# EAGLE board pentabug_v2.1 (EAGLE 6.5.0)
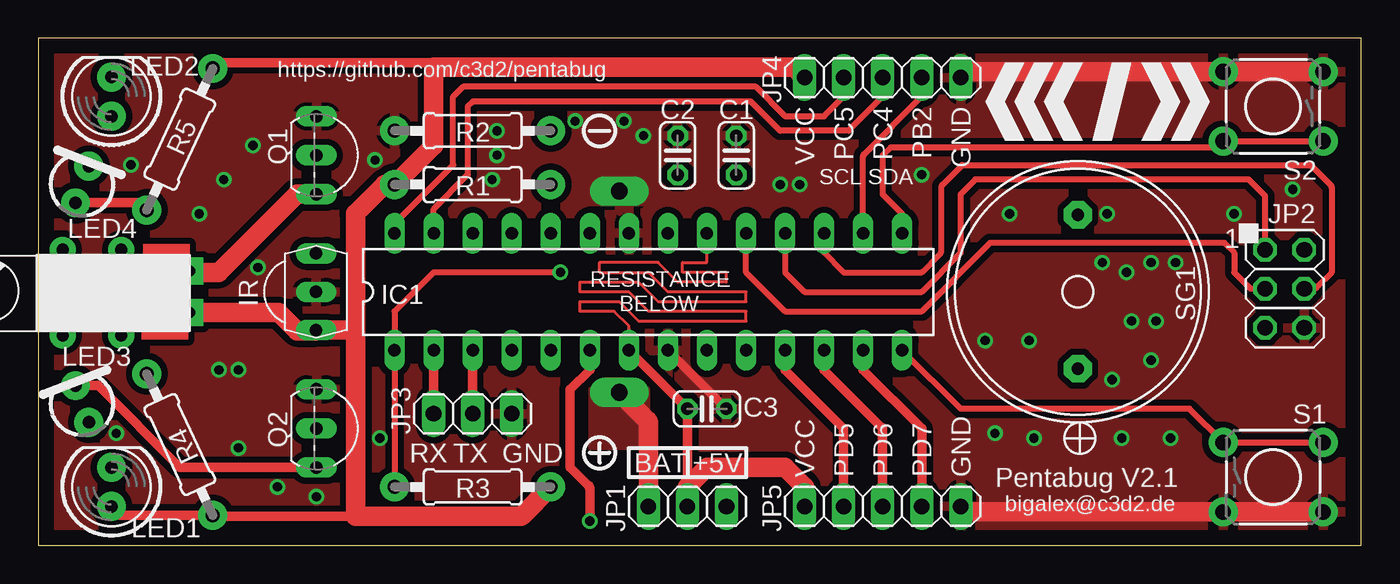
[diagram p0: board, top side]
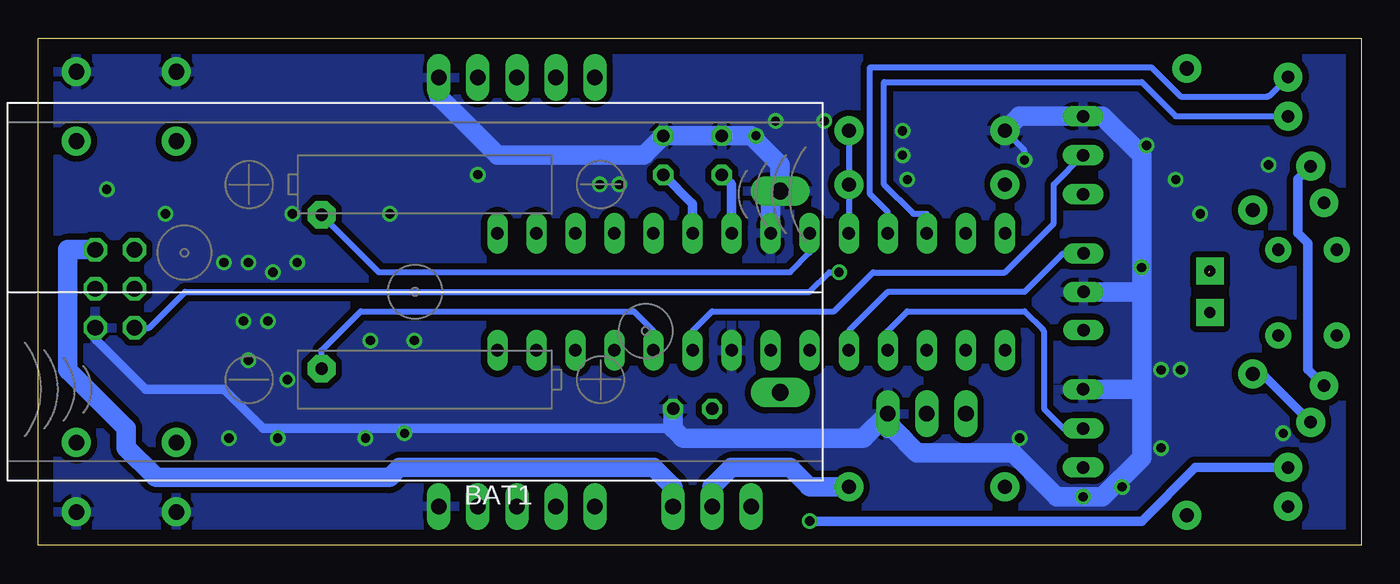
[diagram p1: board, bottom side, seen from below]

Size 86.03 x 33 mm. Coordinates in mm from the lower left corner, seen from the top.
Outline: 86.03,0 86.03,33 0,33 0,0 86.03,0
Copper layers (1*16): Top 0.035mm / dielectric 1.5mm / Bottom 0.035mm
Design rules "default *": minimum track width 8mil, minimum drill 0.6mm, track to track 8mil, track to pad 8mil, pad to pad 8mil, via to via 8mil, smd to smd 8mil, copper to edge 40mil, drill to drill 8mil, minimum pad ring 10mil, minimum via ring 8mil, stop-mask expansion 4mil, vias tented up to drill 0.8mm, thermal gap 10mil

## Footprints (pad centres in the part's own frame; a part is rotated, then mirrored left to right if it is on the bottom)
BATTERY_2XAAA_SMALLPINS = drill 1.1 pad 1.905 long: + -23.75,6.55; - -23.75,-6.55
C025-024X044 = drill 0.813 octagon: 1 -1.27,0; 2 1.27,0
DIL28-3 = drill 0.813 long: 1 -16.51,-3.81; 2 -13.97,-3.81; 3 -11.43,-3.81; 4 -8.89,-3.81; 5 -6.35,-3.81; 6 -3.81,-3.81; 7 -1.27,-3.81; 8 1.27,-3.81; 9 3.81,-3.81; 10 6.35,-3.81; 11 8.89,-3.81; 12 11.43,-3.81; 13 13.97,-3.81; 14 16.51,-3.81; 15 16.51,3.81; 16 13.97,3.81; 17 11.43,3.81; 18 8.89,3.81; 19 6.35,3.81; 20 3.81,3.81; 21 1.27,3.81; 22 -1.27,3.81; 23 -3.81,3.81; 24 -6.35,3.81; 25 -8.89,3.81; 26 -11.43,3.81; 27 -13.97,3.81; 28 -16.51,3.81
TSOP382 = drill 0.813 long: GND -0.001,-0.027; OUT -2.501,-0.027; VCC 2.499,-0.027
1X03 = drill 1.016 long: 1 -2.54,0; 2 0,0; 3 2.54,0
2X03 = drill 1.016 octagon: 1 -2.54,-1.27; 2 -2.54,1.27; 3 0,-1.27; 4 0,1.27; 5 2.54,-1.27; 6 2.54,1.27
1X05 = drill 1.016 long: 1 -5.08,0; 2 -2.54,0; 3 0,0; 4 2.54,0; 5 5.08,0
LED5MM = drill 0.813 pad 1.88: A -1.27,0; K 1.27,0
LED3MM = drill 0.813 pad 1.88: A -1.27,0; K 1.27,0
TO92- = drill 0.813 long: 1 -2.54,0; 2 0,0; 3 2.54,0
0207/10 = drill 0.914 pad 1.88: 1 -5.08,0; 2 5.08,0
TACTILE-PTH = drill 1.016 pad 1.88: 1 -3.251,2.261; 2 3.251,2.261; 3 -3.251,-2.261; 4 3.251,-2.261
BUZZRTDK = drill 0.8 pad 1.8 octagon: + 5,0; - -5,0
LA4-432 = drill 0.7 pad 1.778 square: P$1 -6.985,1.35; P$2 -6.985,-1.35

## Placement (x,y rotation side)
BAT1  BATTERY_2XAAA  [BATTERY_2XAAA_SMALLPINS]  61.53,16.51 180 bottom
C1  100nF  [C025-024X044]  45.39,25.4 270 top
C2  100nF  [C025-024X044]  41.58,25.4 270 top
C3  100nF  [C025-024X044]  43.48,8.89 180 top
IC1  ATMEGA328P-PU  [DIL28-3]  39.67,16.51 0 top
IR  TSOP382  [TSOP382]  18.09,16.51 270 top
JP1  [1X03]  42.21,2.54 180 top
JP2  [2X03]  81.07,16.71 270 top
JP3  [1X03]  28.25,8.57 0 top
JP4  [1X05]  54.91,30.45 0 top
JP5  [1X05]  54.91,2.54 0 top
LED1  [LED5MM]  4.75,3.81 90 top
LED2  [LED5MM]  4.75,29.21 90 top
LED3  [LED3MM]  2.85,9.21 110 top
LED4  [LED3MM]  2.85,23.5 70 top
Q1  [TO92-]  18.09,25.4 270 top
Q2  [TO92-]  18.09,7.62 270 top
R1  100K  [0207/10]  28.25,23.5 0 top
R2  22K  [0207/10]  28.25,26.99 180 top
R3  10k  [0207/10]  28.25,3.81 0 top
R4  33R  [0207/10]  9.2,6.57 295 top
R5  33R  [0207/10]  9.2,26.44 65 top
S1  [TACTILE-PTH]  80.31,4.45 0 top
S2  [TACTILE-PTH]  80.31,28.57 180 top
SG1  MULTIBUZZRTDKBUZZR  [BUZZRTDK]  67.61,16.51 270 top
U$1  VIBRAMOTOR  [LA4-432]  2.85,16.51 180 top

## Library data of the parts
BAT1 IR SG1 U$1 = buglbr
C1-C3 = resistor
IC1 = atmel; OC_FARNELL: unknown; OC_NEWARK: unknown
JP1-JP5 = pinhead
LED1-LED4 S1 S2 = SparkFun
Q1 Q2 R1-R5 = bigalexeasysolder

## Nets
+5V: JP1.1 JP2.2
BAT: BAT1.+ JP1.3
BATLVL: IC1.24 R1.2 R2.1
BUZGND: IC1.23 SG1.-
BUZZR: IC1.10 SG1.+
GND: BAT1.- C1.1 C2.1 C3.1 IC1.8 IC1.22 IR.GND JP2.6 JP3.3 JP4.5 JP5.5 Q1.1 Q2.1 R2.2 S1.3 S1.4 S2.3 S2.4
IRREC: IC1.5 IR.OUT
IRSEND: IC1.4 Q2.2
MISO: IC1.18 JP2.1
MOSI: IC1.17 JP2.4
N$3: IC1.26 LED2.A
N$5: IC1.25 LED2.K
N$7: LED4.A R5.1
N$8: Q1.3 U$1.P$2
N$10: LED3.A R4.1
N$11: LED3.K LED4.K Q2.3
N$12: IC1.6 LED1.K
N$17: C2.2 IC1.21
PB2: IC1.16 JP4.4
PC4/SDA: IC1.27 JP4.3
PC5/SCL: IC1.28 JP4.2
PD5: IC1.11 JP5.2
PD6: IC1.12 JP5.3
PD7: IC1.13 JP5.4
RST: IC1.1 JP2.5 R3.1
RX: IC1.2 JP3.1
S1: IC1.14 S1.1 S1.2
S2: IC1.15 S2.1 S2.2
SCK: IC1.19 JP2.3
TX: IC1.3 JP3.2
VCC: C1.2 C3.2 IC1.7 IC1.20 IR.VCC JP1.2 JP4.1 JP5.1 LED1.A R1.1 R3.2 R4.2 R5.2 U$1.P$1
VIBRATE: IC1.9 Q1.2

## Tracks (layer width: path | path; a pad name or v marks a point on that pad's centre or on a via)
+5V
  Bottom 1.27: JP2.2 84.12,19.25 84.12,11.54 arc-45 84.05,11.36 80.39,7.69 arc45 80.31,7.51 80.31,6.35 78.48,4.52 arc-45 78.3,4.45 63.27,4.45 arc-45 63.1,4.52 62.53,5.08 46.02,5.08 44.83,3.88 arc45 44.75,3.71 JP1.1
BAT
  Top 1.27: BAT1.+ 39.6,8.14 arc-45 39.67,7.96 JP1.3
  pour Top (no thermals): 36.82,10.79 35.86,10.16 35.86,6.35 39.67,6.35 39.67,10.16 38.09,10.79
BATLVL
  Bottom 0.406: R2.1 R1.2 IC1.24
BUZGND
  Bottom 0.406: IC1.23 35.86,19.05 37.13,17.78 63.88,17.78 SG1.-
BUZZR
  Bottom 0.406: SG1.+ 67.61,12.7 65.08,15.24 47.29,15.24 46.02,13.97 IC1.10
GND  (via drill 0.6)
  Top 0.61: IC1.8 C3.1
  Top 1.27: JP4.5 60.31,30.76 arc-45 60.49,30.84 S2.4 S2.3 | S1.4 S1.3 60.46,2.18 arc-45 60.28,2.26 JP5.5
  Bottom 0.406: v21.89,25.08 21.89,25.61 arc-45 21.97,25.79 R2.2
  Bottom 0.61: 44.75,7.62 71.42,7.62 73.89,10.09 arc-45 74.07,10.16 79.05,10.16 82.26,13.38 arc45 82.34,13.56 JP2.6
  Bottom 1.27: IC1.22 38.4,22.44 BAT1.- 37.78,24.78 39.67,26.67 C2.1 C1.1 46.59,25.47 arc45 46.76,25.4 56.18,25.4 59.92,29.14 arc45 59.99,29.32 JP4.5 | 14.28,16.51 14.28,25.4 16.82,27.94 Q1.1 22.21,27.94 R2.2 | C3.1 44.75,7.62 44.19,7.06 arc-45 44.01,6.99 32.48,6.99 arc-45 32.3,7.06 JP3.3 30.79,7.62 30.57,7.62 arc45 30.39,7.55 28.88,6.03 22.64,6.03 19.78,3.17 16.82,3.17 14.28,5.71 14.28,10.16 | IR.GND 14.28,16.51 | 14.28,16.51 14.28,10.16 | Q2.1 14.28,10.16
  other vias: 29.83,25.4 29.83,26.99 29.52,23.81 34.91,27.62 57.45,24.13 38.09,27.62 39.36,26.67 48.25,23.5 49.52,23.5 63.17,21.59 69.52,21.59 81.58,23.18 77.77,21.59 73.97,18.41 72.38,18.41 70.79,17.78 69.2,18.41 72.69,14.61 71.11,14.61 64.44,13.34 61.58,13.34 72.38,12.06 69.84,10.79 62.22,7.3 64.76,6.99 70.47,6.99 73.65,6.99 18.09,3.17 15.55,3.81 13.01,6.35 11.73,11.43 13.01,11.43 14.28,18.1 10.46,21.59 12.05,23.81 13.96,26.04 6.02,24.77 5.07,7.3 22.21,6.99
  pour Top (isolate 0.406, rank 2): -0.96,0 -0.96,34.29 86.03,34.29 86.03,0
  pour Bottom (isolate 0.406): -0.96,0 -0.96,34.29 86.03,34.61 86.03,0.32
  pour Top (no thermals): 35.55,22.23 39.99,22.23 39.99,24.13 38.4,25.4 35.55,25.4
IRREC
  Bottom 0.406: IC1.5 33.32,13.87 arc45 33.25,14.04 30.86,16.44 arc45 30.68,16.51 21.89,16.51 19.47,18.94 arc45 19.29,19.01 IR.OUT
IRSEND
  Bottom 0.406: IC1.4 30.79,13.97 29.52,15.24 21.89,15.24 20.7,14.04 arc45 20.62,13.87 20.62,8.89 19.36,7.62 Q2.2
MISO
  Top 0.406: IC1.18 48.56,17.78 49.83,16.51 57.45,16.51 59.99,19.05 59.99,22.86 60.95,23.81 78.73,23.81 79.8,22.74 JP2.1
MOSI
  Top 0.406: IC1.17 51.1,19.05 52.38,17.78 57.45,17.78 58.65,18.98 arc45 58.72,19.16 58.72,23.29 arc-45 58.8,23.46 60.1,24.77 82.75,24.77 84.05,23.46 arc-45 84.12,23.29 84.12,17.78 83.13,16.78 arc-45 82.95,16.71 JP2.4
N$1  (via drill 0.8 pad 1.68)
  other vias: 1.58,19.25
N$2  (via drill 0.8 pad 1.68)
  other vias: 5.38,19.25
N$3
  Bottom 0.406: IC1.26 28.25,21.59 29.13,21.59 31.04,23.5 31.04,30.16 14.28,30.16 12.05,27.94 LED2.A
N$4  (via drill 0.8 pad 1.68)
  other vias: 5.38,13.67
N$5
  Bottom 0.406: IC1.25 30.79,21.71 31.93,22.86 31.93,31.11 13.64,31.11 11.73,29.21 6.12,29.21 arc-45 5.95,29.28 LED2.K
N$6  (via drill 0.8 pad 1.68)
  other vias: 1.58,13.67
N$7
  Top 0.61: R5.1 6.58,22.3 LED4.A
N$8  (1 unrouted)
  Top 1.27: 9.91,17.78 11.73,17.78 16.82,22.86 Q1.3
N$10
  Bottom 0.61: R4.1 6.44,11.17 LED3.A
N$11
  Top 0.61: LED3.K 3.87,10.4 9.2,5.08 Q2.3
  Bottom 0.61: LED4.K 4.12,23.85 4.12,20.32 3.48,19.68 3.48,11.47 LED3.K
N$12  (via drill 0.6)
  Top 0.61: IC1.6 35.86,11.43 34.59,10.16 34.59,5.08 35.79,3.88 arc-45 35.86,3.71 v35.86,1.59
  Bottom 0.61: v35.86,1.59 14.28,1.59 10.78,5.08 LED1.K
N$17
  Bottom 0.61: C2.2 41.02,23.57 arc45 40.94,23.39 IC1.21
PB2
  Top 0.406: IC1.16 53.64,25.3 arc-45 53.72,25.47 57.38,29.14 arc45 57.45,29.32 JP4.4
PC4/SDA
  Top 0.406: JP4.3 54.91,29.21 52.69,26.99 48.25,26.99 46.34,28.89 28.25,28.89 27.93,28.57 27.93,24.13 25.71,21.91 IC1.27
PC5/SCL
  Top 0.406: JP4.2 52.38,29.21 51.1,27.94 48.56,27.94 46.66,29.84 27.61,29.84 26.98,29.21 26.98,24.77 23.16,20.95 IC1.28
PD5
  Top 0.61: IC1.11 48.56,11.43 52.38,7.62 JP5.2
PD6
  Top 0.61: IC1.12 51.1,11.43 54.84,7.69 arc-45 54.91,7.51 JP5.3
PD7
  Top 0.61: IC1.13 53.64,11.43 57.45,7.62 JP5.4
RST  (via drill 0.6)
  Top 0.406: v33.96,17.78 25.71,17.78 23.16,15.24 IC1.1 R3.1
  Bottom 0.406: JP2.5 78.84,14.17 76.5,16.51 35.86,16.51 34.59,17.78 v33.96,17.78
RX
  Top 0.61: JP3.1 IC1.2
S1
  Top 0.406: S1.2 S1.1 74.88,8.89 59.99,8.89 IC1.14
S2
  Top 0.406: S2.1 S2.2 76.67,25.92 55.44,25.92 54.91,25.4 54.91,22.86 56.18,21.59 IC1.15
SCK
  Top 0.406: IC1.19 46.02,17.78 48.56,15.24 57.45,15.24 61.9,19.68 77.14,19.68 77.77,19.05 77.77,17.78 78.84,16.71 JP2.3
TX
  Top 0.61: JP3.2 IC1.3
VCC
  Top 0.203: IC1.7 38.4,14.29 37.45,15.24 35.23,15.24 35.23,15.88 37.77,15.88 39.04,14.61 46.02,14.61 46.02,15.24 39.67,15.24 38.4,16.51 35.23,16.51 35.23,17.14 39.04,17.14 40.31,15.88 46.02,15.88 46.02,16.51 40.94,16.51 39.67,17.78 36.5,17.78 36.5,18.41 40.31,18.41 41.58,17.14 44.75,17.14 44.75,17.78 41.9,17.78 41.9,18.41 43.48,18.41 IC1.20
  Top 0.61: IC1.7 C3.2 42.21,3.81 | 25.71,31.11 25.39,31.43 11.73,31.43 R5.2 | 20.62,1.91 11.4,1.91 R4.2 5.32,1.97 LED1.A
  Top 1.27: U$1.P$1 15.62,15.16 16.82,13.97 18.02,13.97 IR.VCC 20.58,14.01 20.62,13.97 | JP5.1 49.83,3.81 48.56,5.08 43.48,5.08 42.21,3.81 JP1.2 | 20.62,13.97 20.62,21.59 22.53,23.5 R1.1 25.71,26.04 25.71,31.11 49.17,31.11 JP4.1 | 20.62,13.97 20.62,1.91 31.32,1.91 arc45 31.49,1.98 33.25,3.74 arc45 33.32,3.92 R3.2
  Bottom 0.61: IC1.20 43.48,22.12 arc-45 43.56,22.3 C1.2
  Bottom 1.27: 42.21,3.81 JP1.2 42.21,3.71 arc45 42.14,3.88 40.94,5.08 37.13,5.08 35.94,3.88 arc-45 35.76,3.81 R3.2
VIBRATE
  Bottom 0.406: IC1.9 43.48,13.97 42.21,15.24 34.28,15.24 31.74,17.78 23.16,17.78 19.99,20.95 19.99,23.5 Q1.2

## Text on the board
tNames: https://github.com/c3d2/pentabug | VCC | PC5 | PC4 | PB2 | GND | SCL | SDA | 1 | RESISTANCE | IR | BELOW | RX | TX | GND | BAT | +5V | VCC | PD5 | PD6 | PD7 | GND | Pentabug V2.1 | bigalex@c3d2.de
